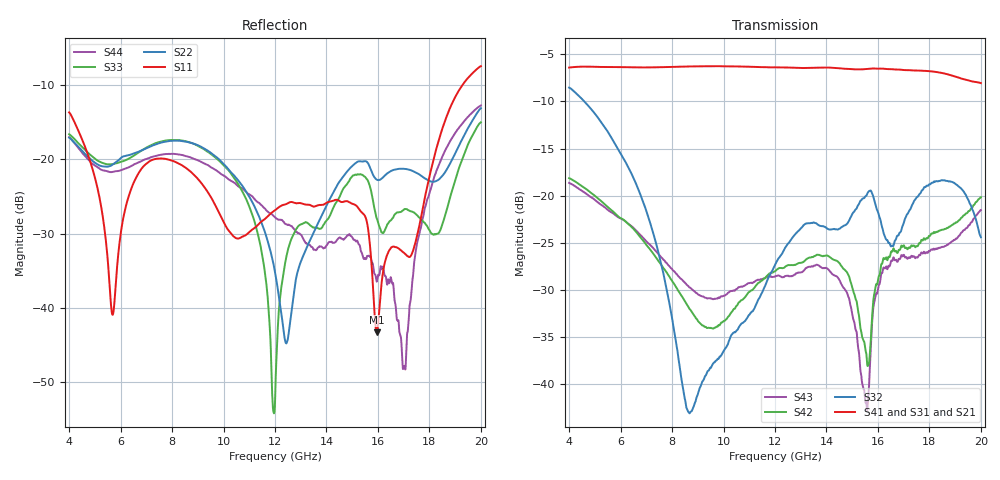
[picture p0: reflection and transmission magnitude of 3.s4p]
!Keysight Technologies,N5247B,US57180241,A.12.85.04
!Date: Friday, March 23, 2018 09:49:27
!Correction: S11(Full 4 Port(1,2,3,4))
!S12(Full 4 Port(1,2,3,4))
!S13(Full 4 Port(1,2,3,4))
!S14(Full 4 Port(1,2,3,4))
!S21(Full 4 Port(1,2,3,4))
!S22(Full 4 Port(1,2,3,4))
!S23(Full 4 Port(1,2,3,4))
!S24(Full 4 Port(1,2,3,4))
!S31(Full 4 Port(1,2,3,4))
!S32(Full 4 Port(1,2,3,4))
!S33(Full 4 Port(1,2,3,4))
!S34(Full 4 Port(1,2,3,4))
!S41(Full 4 Port(1,2,3,4))
!S42(Full 4 Port(1,2,3,4))
!S43(Full 4 Port(1,2,3,4))
!S44(Full 4 Port(1,2,3,4))
!S4P File: Measurements: <S11,S12,S13,S14>,
!<S21,S22,S23,S24>,
!<S31,S32,S33,S34>,
!<S41,S42,S43,S44>:
# Hz S  dB  R 50
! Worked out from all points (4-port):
!   6401 points, 4 GHz to 20 GHz, reference 50 ohm
!   strongest paths, dB at 4 GHz, 8 GHz, 12 GHz, 16 GHz, 20 GHz:
!     S41: -6.4, -6.3, -6.4, -6.5, -8.1
!     S31: -6.5, -6.3, -6.5, -6.7, -7.9
!     S21: -6.4, -6.5, -6.6, -6.2, -8.4
!     S32: -8.5, -33.0, -27.4, -21.7, -24.4
!     S42: -18.1, -29.0, -28.0, -29.0, -20.2
!     S43: -18.6, -27.8, -28.6, -30.0, -21.5
!   lowest |S11| = -43.3 dB at 15.95 GHz (marker M1), VSWR 1.01, Z = 50.6 - j0.308 ohm
!   |S11| at or under -10 dB: start of sweep to 19.29 GHz
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4e9  -13.71 22.7  -6.46 -147.8  -6.55 -149.4  -6.40 -148.7
     -6.41 -147.6  -17.10 -22.7  -8.53 -120.4  -18.11 122.0
     -6.50 -149.4  -8.53 -120.6  -16.65 -24.2  -18.60 120.7
     -6.40 -148.8  -18.15 121.6  -18.65 120.6  -17.04 -22.3
5.6875e9  -40.91 39.3  -6.22 143.0  -6.27 141.3  -6.32 142.0
          -6.20 143.2  -20.74 -33.3  -14.04 -173.0  -21.60 27.6
          -6.26 141.3  -14.05 -173.1  -20.65 -39.9  -21.81 22.6
          -6.35 141.9  -21.64 27.4  -21.84 22.5  -21.71 -34.3
8.6775e9  -21.55 -32.8  -6.50 19.0  -6.38 17.5  -6.26 18.8
          -6.45 19.0  -17.74 -95.0  -43.16 -164.4  -31.95 -177.3
          -6.31 17.1  -43.11 -165.0  -17.73 -96.6  -29.65 176.1
          -6.28 18.8  -32.03 -177.3  -29.76 176.5  -19.72 -104.4
1.1945e10  -27.00 60.4  -6.53 -123.9  -6.45 -126.0  -6.32 -124.3
           -6.58 -123.8  -34.16 171.9  -27.68 -72.3  -28.09 -102.1
           -6.47 -126.3  -27.67 -72.7  -54.02 97.4  -28.58 -85.6
           -6.38 -124.1  -28.10 -102.0  -28.61 -85.1  -27.64 105.5
1.595e10  -43.25 -26.3  -6.21 41.2  -6.89 42.1  -6.65 43.5
          -6.13 41.4  -22.74 -70.2  -21.59 -161.8  -29.47 67.6
          -6.65 42.5  -21.43 -161.6  -27.94 -96.7  -30.31 79.9
          -6.51 44.1  -29.42 68.0  -30.40 80.1  -36.46 150.0
1.70225e10  -32.62 -48.8  -6.90 -14.4  -7.02 -13.0  -6.69 -12.3
            -7.00 -14.2  -21.30 -91.3  -22.93 -136.3  -25.49 -15.2
            -6.86 -13.8  -22.67 -137.3  -26.73 -72.0  -26.22 -12.4
            -6.67 -12.2  -25.37 -15.3  -26.37 -11.5  -47.98 106.1
2e10  -7.50 55.9  -8.11 178.6  -7.97 -177.0  -8.07 -175.1
      -8.38 178.2  -13.15 62.8  -24.73 152.1  -20.45 154.4
      -7.91 -179.4  -24.41 150.0  -15.04 49.2  -21.52 151.5
      -8.05 -176.9  -20.17 153.1  -21.53 152.0  -12.78 56.8
